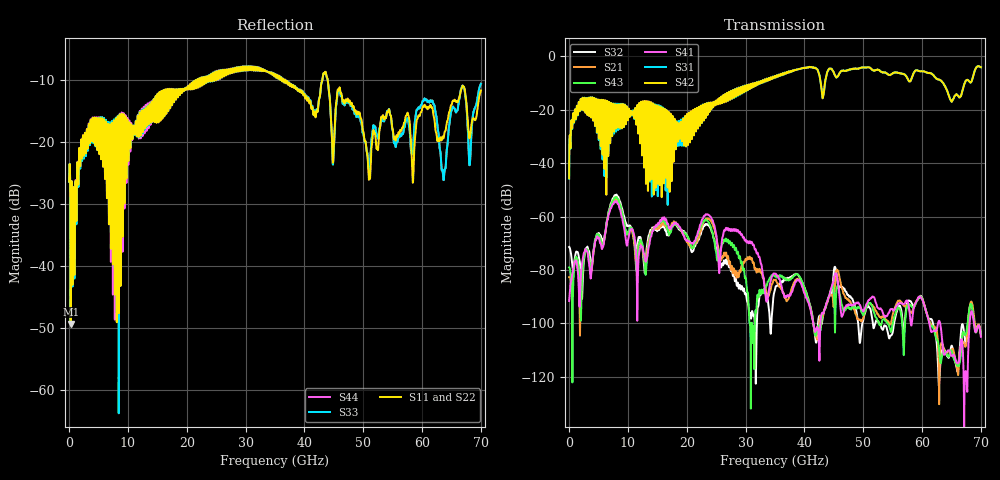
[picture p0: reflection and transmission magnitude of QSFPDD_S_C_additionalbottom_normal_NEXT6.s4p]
! AWR Design Environment (8415) Thu Dec 20 14:48:39 2018
! Document = 'CHANNEL TEST'
! nPorts: 4, nXvals: 7001
# HZ S DB R 50
!Freq DBS11 AngS11 DBS12 AngS12 DBS13 AngS13 DBS14 AngS14
!	DBS21 AngS21 DBS22 AngS22 DBS23 AngS23 DBS24 AngS24
!	DBS31 AngS31 DBS32 AngS32 DBS33 AngS33 DBS34 AngS34
!	DBS41 AngS41 DBS42 AngS42 DBS43 AngS43 DBS44 AngS44
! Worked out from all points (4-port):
!   7000 points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, 10 MHz to 70 GHz, reference 50 ohm
!   strongest paths, dB at 10 MHz, 17.51 GHz, 35.01 GHz, 52.51 GHz, 70 GHz:
!     S42: -45.6, -25.5, -7.4, -5.0, -4.0
!     S31: -45.8, -26.2, -7.4, -5.0, -4.0
!     S41: -91.6, -63.2, -81.5, -94.2, -105.0
!     S43: -79.0, -63.9, -82.5, -99.0, -104.1
!     S21: -82.7, -62.3, -83.7, -96.6, -104.5
!     S32: -71.4, -62.8, -87.2, -99.2, -103.7
!   lowest |S11| = -49.4 dB at 270 MHz (marker M1), VSWR 1.01, Z = 49.7 - j0.103 ohm
!   |S11| at or under -10 dB: start of sweep to 21.8 GHz; 36.46 GHz to 43.06 GHz (6.604 GHz wide, 16.6 % of centre); 43.96 GHz to end of sweep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
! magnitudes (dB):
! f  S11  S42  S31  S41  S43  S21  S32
! 10 MHz  -26.5  -45.6  -45.8  -91.6  -79.0  -82.7  -71.4
! 270 MHz  -49.4  -31.0  -31.2  -85.0  -81.3  -83.5  -73.1
! 7.98 GHz  -16.6  -27.0  -27.9  -54.4  -52.8  -53.5  -51.9
! 12.85 GHz  -17.8  -17.8  -18.2  -75.1  -77.6  -77.3  -80.9
! 23.49 GHz  -9.4  -20.4  -20.3  -59.2  -61.5  -60.7  -62.8
! 28.1 GHz  -8.5  -13.9  -14.0  -65.0  -71.4  -81.2  -82.8
! 70 GHz  -11.8  -4.0  -4.0  -105.0  -104.1  -104.5  -103.7
